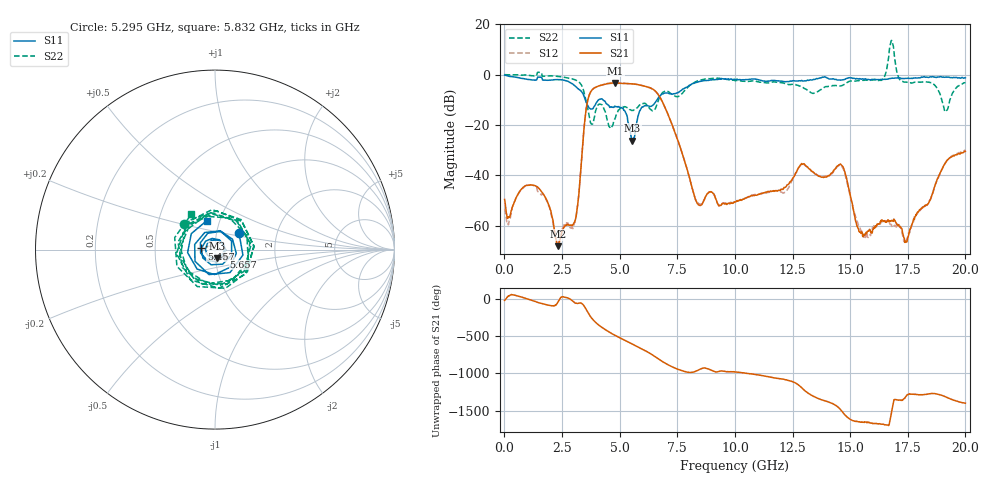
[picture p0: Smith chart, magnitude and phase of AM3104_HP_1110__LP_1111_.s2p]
!Created with skrf (http://scikit-rf.org).
# Hz S RI R 50.0
!freq ReS11 ImS11 ReS21 ImS21 ReS12 ImS12 ReS22 ImS22
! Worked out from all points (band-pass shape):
!   1601 points, 10 MHz to 20 GHz, reference 50 ohm
!   highest |S21| = -3.34 dB at 4.808 GHz (marker M1); lowest = -68.1 dB at 2.321 GHz (marker M2)
!   |S21| within 3 dB of the highest: 3.787 GHz to 6.52 GHz (2.733 GHz wide, 53 % of centre)
!   lowest |S11| = -26.2 dB at 5.545 GHz (marker M3), VSWR 1.10, Z = 51 - j4.86 ohm
!   |S11| at or under -10 dB: 3.512 GHz to 4.1 GHz (588.2 MHz wide, 15.5 % of centre); 4.272 GHz to 6.627 GHz (2.355 GHz wide, 43.2 % of centre)
!   |S22| runs from -21.4 to 13.5 dB; largest |S21 - S12| = 0.081
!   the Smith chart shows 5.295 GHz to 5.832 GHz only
!   S11 on the Smith chart (normalised r, x): 5.295 GHz: 1.29, +0.24; 5.457 GHz: 0.86, +0.01; 5.657 GHz: 1.10, -0.08; 5.832 GHz: 0.87, +0.29
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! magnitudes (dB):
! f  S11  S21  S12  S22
! 10 MHz  -0.2  -49.5  -53.3  -0.1
! 1.297 GHz  -2.2  -44.0  -44.2  -0.6
! 2.321 GHz  -2.0  -68.1  -67.1  -0.8
! 3.033 GHz  -4.3  -58.6  -59.1  -2.0
! 3.346 GHz  -6.8  -34.1  -34.1  -4.2
! 3.721 GHz  -13.6  -7.3  -7.3  -18.5
! 4.808 GHz  -12.6  -3.3  -3.4  -17.4
! 5.295 GHz  -15.8  -3.5  -3.6  -13.0
! 5.457 GHz  -22.4  -3.6  -3.6  -13.9
! 5.545 GHz  -26.2  -3.7  -3.7  -14.2
! 5.657 GHz  -24.2  -3.8  -3.8  -14.0
! 5.832 GHz  -15.5  -4.1  -4.1  -12.5
! 6.682 GHz  -9.2  -8.0  -8.0  -10.2
! 8.381 GHz  -3.0  -51.3  -50.8  -2.5
! 10.01 GHz  -2.0  -50.6  -50.6  -2.4
! 13.34 GHz  -2.2  -38.4  -38.5  -7.4
! 14.65 GHz  -2.2  -36.2  -36.6  -4.4
! 15.49 GHz  -1.8  -62.8  -62.1  -2.4
! 16.68 GHz  -1.7  -58.0  -58.5  7.2
! 17.45 GHz  -1.5  -66.5  -65.7  -3.1
! 19.16 GHz  -1.0  -34.5  -34.6  -14.4
! 20 GHz  -1.3  -30.5  -30.0  -3.2
